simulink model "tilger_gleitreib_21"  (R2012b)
settings: Solver=ode23  StartTime=0.0  StopTime=10.0  FixedStep=dt  MaxStep=dt  RelTol=1e-3
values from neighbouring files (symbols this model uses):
  c2 = 2*m2*sqrt(k2/m2)*sqrt(3*mu/(8*(1+mu)))    [feder_masse_1.m]    (also in feder_masse_13.m; feder_masse_14.m; tilger_gleitreib21.m; vibration_control_1.m = 2*m2*sqrt(k2/m2)*sqrt(3*mu/(8*(1+mu))),)
  dt = 0.001    [coulomb_1.m]    (also in coulomb_10.m; coulomb_11.m; coulomb_2.m; coulomb_3.m)
  Fex_ampl = 800    [coulomb_1.m]    (also in coulomb_2.m; coulomb_3.m; coulomb_4.m; coulomb_5.m)
  k1 = 5000    [feder_masse_1.m]    (also in feder_masse_11.m; feder_masse_13.m; feder_masse_14.m; tilger_gleitreib21.m)
  k2 = mu*k1/((1+mu)^2)    (= 226.757369615)    [feder_masse_1.m]    (also in feder_masse_13.m; feder_masse_14.m; tilger_gleitreib21.m; unwucht_synchro1.m = 5e-05)
  m1 = 100    [feder_masse_1.m]    (also in feder_masse_11.m; feder_masse_13.m; feder_masse_14.m; position_reg_2.m = 1)
  m2 = 5    [feder_masse_1.m]    (also in feder_masse_13.m; feder_masse_14.m; foerd_gleit_1.m = 0.1; tilger_gleitreib21.m)
  rg = 20    [tilger_gleitreib1.m]    (also in tilger_gleitreib2.m = 100; tilger_gleitreib21.m = 0.5; tilger_gleitreib3.m = 8,      m1 = 0.1)
  v0 = 0    [coulomb_1.m]    (also in coulomb_2.m; coulomb_3.m; coulomb_4.m; coulomb_5.m)
  v02 = 0    [tilger_gleitreib21.m]
  w01 = sqrt(k1/m1)    [feder_masse_1.m]    (also in feder_masse_11.m; feder_masse_12.m = 0.12; tilger_gleitreib21.m; vibration_control_1.m = sqrt(k1/m1),      w02 = sqrt(k2/m2),)
  y0 = 0    [coulomb_1.m]    (also in coulomb_2.m; coulomb_3.m; coulomb_4.m; coulomb_5.m)
  y02 = 0    [tilger_gleitreib21.m]

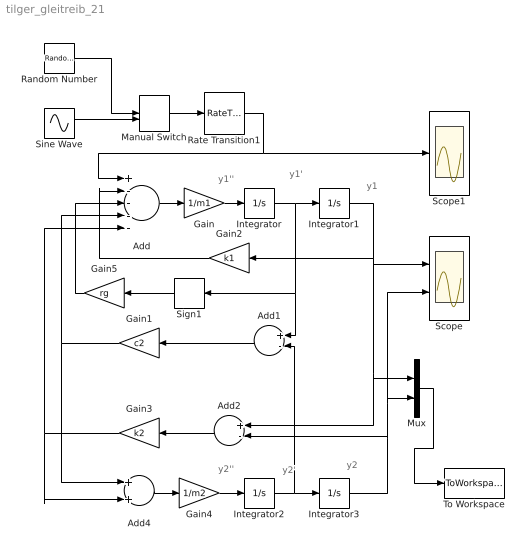
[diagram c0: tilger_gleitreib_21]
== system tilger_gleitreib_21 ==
  note: y1'
  note: y2
  note: y1
  note: y1''
  note: y2'
  note: y2''
  Add : Sum  Inputs=+----
  Add1 : Sum  Inputs=+-
  Add2 : Sum  Inputs=+-
  Add4 : Sum
  Gain : Gain  Gain=1/m1
  Gain1 : Gain  Gain=c2
  Gain2 : Gain  Gain=k1
  Gain3 : Gain  Gain=k2
  Gain4 : Gain  Gain=1/m2
  Gain5 : Gain  Gain=rg
  Integrator : Integrator  InitialCondition=v0
  Integrator1 : Integrator  InitialCondition=y0
  Integrator2 : Integrator  InitialCondition=v02
  Integrator3 : Integrator  InitialCondition=y02
  Manual Switch : ManualSwitch  CurrentSetting=0
  Mux : Mux  Inputs=2
  Random Number : RandomNumber  Variance=Fex_ampl  SampleTime=100*dt
  Rate Transition1 : RateTransition  OutPortSampleTime=dt
  Scope : Scope  NumInputPorts=2
  Scope1 : Scope
  Sign1 : Signum  ZeroCross=off
  Sine Wave : Sin  Amplitude=Fex_ampl  Frequency=w01  SampleTime=100*dt
  To Workspace : ToWorkspace  VariableName=y  SampleTime=-1  SaveFormat=Structure With Time
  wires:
  Add/1 -> Gain/1
  Integrator/1 -> Sign1/1, Add1/1, Integrator1/1
  Gain/1 -> Integrator/1
  Gain1/1 -> Add/4, Add4/1
  Add2/1 -> Gain3/1
  Gain4/1 -> Integrator2/1
  Integrator2/1 -> Add1/2, Integrator3/1
  Integrator3/1 -> Scope/2, Mux/2, Add2/2
  Add4/1 -> Gain4/1
  Integrator1/1 -> Scope/1, Add2/1, Mux/1, Gain2/1
  Mux/1 -> To Workspace/1
  Add1/1 -> Gain1/1
  Gain2/1 -> Add/2
  Sign1/1 -> Gain5/1
  Gain5/1 -> Add/3
  Gain3/1 -> Add/5, Add4/2
  Rate Transition1/1 -> Scope1/1, Add/1
  Manual Switch/1 -> Rate Transition1/1
  Random Number/1 -> Manual Switch/1
  Sine Wave/1 -> Manual Switch/2
